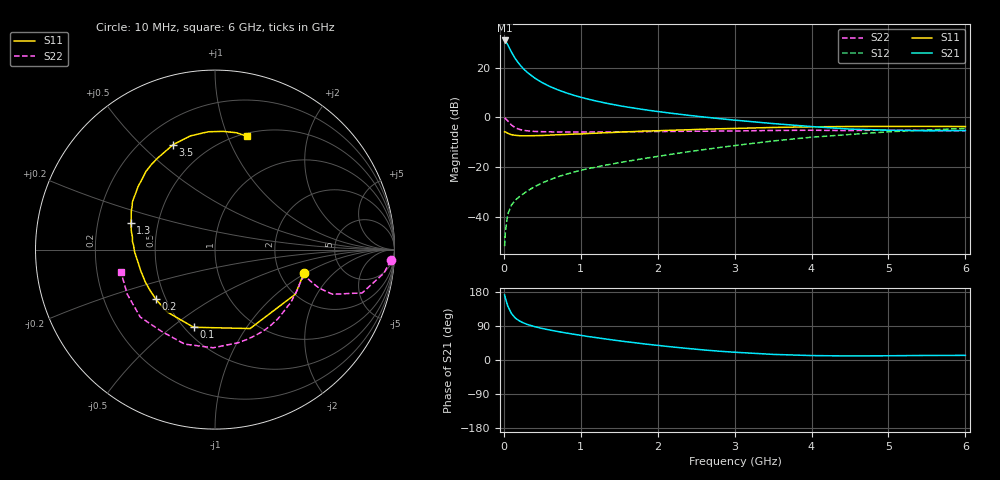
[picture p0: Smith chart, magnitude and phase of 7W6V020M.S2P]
! Infineon Technologies  Discrete & RF Semiconductors
! BFS17W
! Si NPN RF Bipolar Junction Transistor in SOT323
! VCE = 6 V  IC = 20 mA
! Common Emitter S-Parameters:  August  1999
# GHz  S  MA  R  50
!  f  S11  S21  S12  S22
! GHz  MAG  ANG  MAG  ANG  MAG  ANG  MAG  ANG
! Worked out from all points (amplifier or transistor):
!   36 points, 10 MHz to 6 GHz, reference 50 ohm
!   highest |S21| = 30.9 dB at 10 MHz (marker M1)
!   |S21| within 3 dB of that: start of sweep to 71.66 MHz
!   unconditionally stable (mu >= 1): 293.4 MHz to 2.097 GHz; 5.366 GHz to end of sweep
!   at 250 MHz: K = 0.95, MSG = 25.2 dB, |S12| = -30.8 dB
!   at 1.4 GHz: K = 1.15, MAG = 9.7 dB, |S12| = -18.7 dB
!   at 6 GHz: K = 1.04, MAG = -1.7 dB, |S12| = -4.4 dB
!   S11 on the Smith chart (normalised r, x): 10 MHz: 2.72, -0.96; 100 MHz: 0.55, -0.60; 200 MHz: 0.44, -0.30; 1.3 GHz: 0.35, +0.14; 3.5 GHz: 0.32, +0.63; 6 GHz: 0.53, +1.17
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0.01  0.5128 -14.6  35.14 171.7  0.0026 79.0  0.9814 -3.5
0.02  0.5121 -29.0  34.12 163.4  0.0051 82.4  0.9507 -7.9
0.05  0.4814 -66.0  28.94 142.9  0.0113 67.8  0.8547 -16.4
0.1  0.4488 -105.4  20.4 122.3  0.0175 60.6  0.7006 -20.8
0.15  0.4378 -127.4  15.08 110.6  0.0218 59.3  0.6186 -20.3
0.2  0.4302 -140.0  11.83 103.5  0.0255 62.7  0.5776 -19.0
0.25  0.4274 -149.0  9.654 98.3  0.029 62.2  0.5528 -17.9
0.3  0.4281 -155.4  8.144 94.3  0.033 64.2  0.5406 -17.3
0.4  0.4306 -164.4  6.199 88.0  0.0407 65.7  0.5238 -16.9
0.5  0.4343 -170.5  4.989 83.2  0.0486 68.4  0.518 -17.2
0.6  0.4416 -175.1  4.167 79.0  0.0562 69.1  0.5138 -18.1
0.7  0.449 -178.9  3.595 75.2  0.0643 70.3  0.5116 -19.4
0.9  0.4624 174.3  2.814 68.3  0.0791 71.3  0.509 -22.7
1.1  0.4764 167.9  2.321 61.8  0.0943 71.8  0.5107 -26.7
1.3  0.4919 162.3  1.977 56.1  0.1088 72.0  0.5105 -31.1
1.6  0.5151 154.7  1.62 48.0  0.1314 72.9  0.5136 -38.1
2.2  0.5539 140.7  1.202 34.2  0.1844 73.8  0.5242 -53.7
2.8  0.5918 126.8  0.948 23.2  0.2486 71.7  0.5314 -70.6
3.5  0.6295 111.8  0.753 14.8  0.3369 66.3  0.5469 -91.1
4.5  0.6576 93.3  0.583 10.6  0.4553 53.7  0.5443 -123.3
5.5  0.6619 79.7  0.539 12.0  0.5603 40.6  0.5486 -153.0
6  0.6565 74.4  0.547 12.2  0.6019 34.1  0.5385 -166.3
